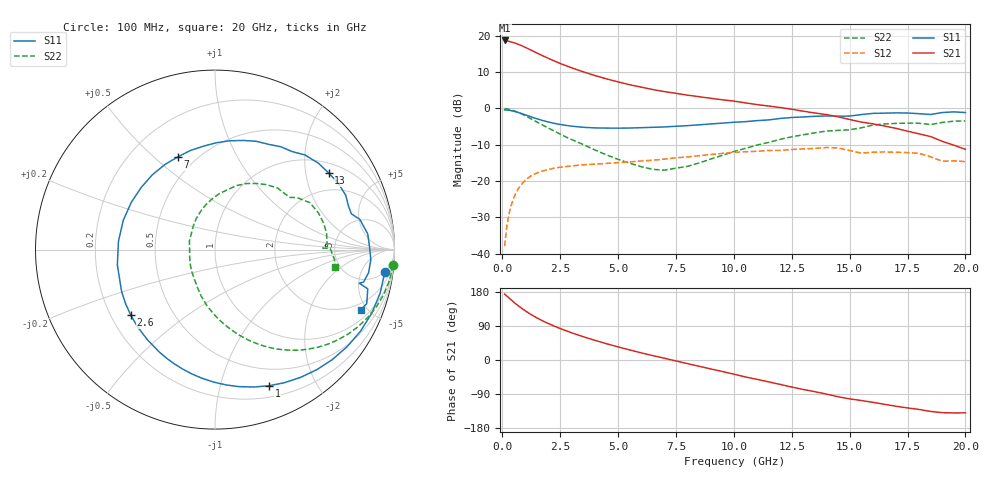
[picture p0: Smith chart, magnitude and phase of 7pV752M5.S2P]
! Infineon Technologies  Discrete & RF Semiconductors
! bfp620
! VCE = 0.75 V,  IC =  2.5 mA
! Common Emitter S-Parameters:  Sep 2002
# GHz  S  MA  R  50
!  f  S11  S21  S12  S22
! GHz  MAG  ANG  MAG  ANG  MAG  ANG  MAG  ANG
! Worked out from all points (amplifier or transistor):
!   59 points, 100 MHz to 20 GHz, reference 50 ohm
!   highest |S21| = 18.7 dB at 100 MHz (marker M1)
!   |S21| within 3 dB of that: start of sweep to 1.348 GHz
!   unconditionally stable (mu >= 1): 5.613 GHz to 13.29 GHz; 14.29 GHz to 15.8 GHz; 17.01 GHz to end of sweep
!   at 1 GHz: K = 0.20, MSG = 18.3 dB, |S12| = -19.7 dB
!   at 5.5 GHz: K = 0.99, MSG = 10.6 dB, |S12| = -14.7 dB
!   at 20 GHz: K = 1.69, MAG = -3.2 dB, |S12| = -14.7 dB
!   S11 on the Smith chart (normalised r, x): 100 MHz: 5, -14; 1 GHz: 0.31, -1.42; 2.6 GHz: 0.28, -0.32; 7 GHz: 0.40, +0.60; 13 GHz: 1.31, +2.69; 20 GHz: 1.54, -4.53
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0.1  0.9544 -7.4  8.638 173.8  0.0127 85.4  0.9956 -5.0
0.3  0.9427 -22.0  8.374 163.2  0.0367 77.5  0.9735 -14.7
0.6  0.8962 -43.1  7.837 147.5  0.0696 65.2  0.9063 -28.2
0.8  0.8571 -56.1  7.401 138.1  0.0878 57.8  0.8503 -36.2
1  0.816 -68.4  6.927 129.5  0.103 51.1  0.7911 -43.4
1.3  0.7566 -85.3  6.221 117.9  0.1205 42.5  0.7036 -52.9
1.7  0.6894 -105.2  5.403 104.6  0.1365 33.4  0.6002 -63.3
2.2  0.6281 -126.7  4.576 90.6  0.1495 24.9  0.4961 -74.1
2.6  0.595 -142.1  4.048 80.7  0.1565 19.4  0.4276 -81.9
3  0.5702 -155.9  3.62 71.7  0.1619 14.6  0.3724 -89.2
3.5  0.5506 -171.2  3.193 61.4  0.1674 9.7  0.3184 -97.8
4  0.5399 175.1  2.838 51.9  0.1712 5.5  0.2686 -106.9
5  0.5356 150.5  2.322 34.5  0.1796 -1.0  0.1992 -125.5
6  0.5438 129.8  1.965 18.9  0.1889 -6.8  0.1576 -151.9
7  0.5564 111.8  1.708 4.7  0.2009 -12.1  0.1414 177.8
8.5  0.5956 89.2  1.452 -16.5  0.2237 -21.7  0.1776 133.4
10.5  0.6584 62.9  1.194 -44.7  0.2538 -38.4  0.2819 93.5
13  0.7637 34.0  0.917 -77.8  0.2774 -59.5  0.4346 58.0
13.5  0.7799 28.4  0.866 -83.6  0.2822 -64.3  0.4618 51.6
15  0.7853 14.7  0.705 -102.6  0.2633 -84.3  0.5094 34.8
17  0.8701 -3.8  0.532 -122.0  0.2491 -94.9  0.6227 13.6
20  0.8783 -22.5  0.274 -139.5  0.1851 -113.6  0.6743 -8.5
